PROGRAM MAIN
VAR
	{attribute 'OPC.UA.DA' := '1'}
	{attribute'OPC.UA.DA.Access' := '1'}
	// Access: 0 => no access, 1 => readonly, 2 => writeonly, 3 (default) => rw
	preklopnik: BOOL;
	{attribute 'OPC.UA.DA' := '1'}
	{attribute'OPC.UA.DA.Access' := '3'} 
	{attribute 'OPC.UA.DA.Description' :='ID izdelka'}
	izdelekID: INT;
	{attribute 'OPC.UA.DA' := '1'}
	recept: ST_recept;
END_VAR

AlarmsAndEvents();
AlarmsAndEventsCX7000();

END_PROGRAM
